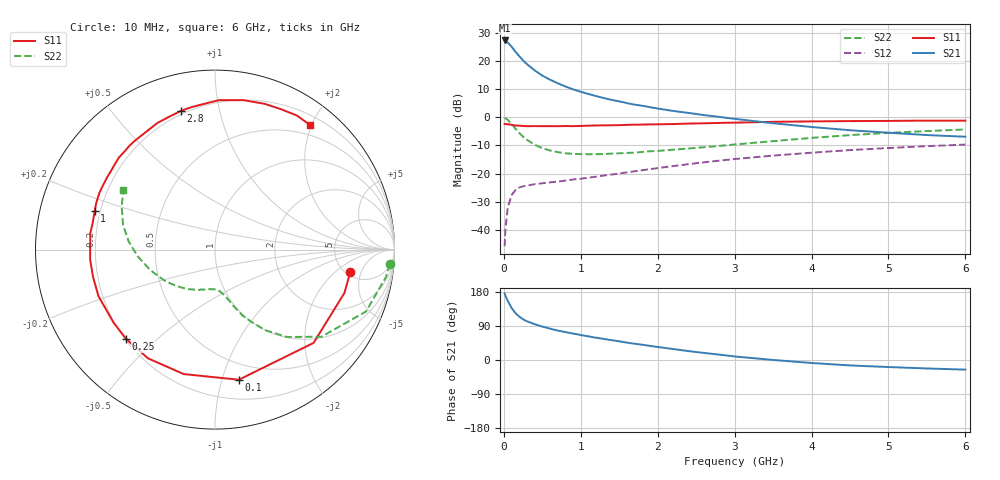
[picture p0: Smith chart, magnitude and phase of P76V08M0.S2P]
! SIEMENS Small Signal Semiconductors
! BFP196
! Si NPN RF Bipolar Junction Transistor in SOT143
! VCE = 6 V  IC = 8 mA
! Common Emitter S-Parameters:  May  1996
# GHz  S  MA  R  50
!  f  S11  S21  S12  S22
! GHz  MAG  ANG  MAG  ANG  MAG  ANG  MAG  ANG
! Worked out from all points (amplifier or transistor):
!   36 points, 10 MHz to 6 GHz, reference 50 ohm
!   highest |S21| = 27.4 dB at 10 MHz (marker M1)
!   |S21| within 3 dB of that: start of sweep to 123.2 MHz
!   unconditionally stable (mu >= 1): 965.9 MHz to 3.225 GHz
!   at 250 MHz: K = 0.34, MSG = 22.4 dB, |S12| = -24.5 dB
!   at 1.4 GHz: K = 1.14, MAG = 11.1 dB, |S12| = -20.4 dB
!   at 6 GHz: K = 0.97, MSG = 1.4 dB, |S12| = -9.7 dB
!   S11 on the Smith chart (normalised r, x): 10 MHz: 5.46, -3.27; 100 MHz: 0.36, -1.14; 250 MHz: 0.20, -0.40; 1 GHz: 0.18, +0.15; 2.8 GHz: 0.18, +0.77; 6 GHz: 0.34, +1.97
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0.01  0.764 -9.4  23.36 175.9  0.0051 88.6  0.9781 -4.8
0.02  0.7605 -18.5  22.82 169.8  0.01 81.9  0.9642 -9.2
0.05  0.7563 -43.4  21.47 156.3  0.0245 68.3  0.9092 -22.3
0.1  0.7371 -79.6  18.21 137.6  0.0412 53.7  0.7663 -39.3
0.15  0.7151 -104.1  14.79 123.8  0.0507 43.7  0.6301 -50.6
0.2  0.7116 -121.6  12.29 114.6  0.0563 37.9  0.5298 -58.0
0.25  0.702 -134.8  10.28 107.4  0.0593 34.2  0.4518 -63.2
0.3  0.6964 -144.2  8.852 102.2  0.0611 32.1  0.3989 -67.3
0.4  0.6991 -158.2  6.865 94.5  0.0646 30.1  0.3258 -72.2
0.5  0.6965 -167.4  5.544 88.2  0.0671 29.6  0.2834 -75.6
0.6  0.698 -175.5  4.679 82.7  0.0697 30.3  0.2569 -78.8
0.7  0.6958 177.8  4.041 77.8  0.0718 31.8  0.2406 -81.9
0.8  0.7008 172.4  3.545 73.7  0.075 32.6  0.2299 -84.6
1  0.7041 162.4  2.849 65.9  0.0809 35.1  0.2218 -89.2
1.1  0.7111 158.5  2.6 62.3  0.0844 36.4  0.2209 -92.2
1.6  0.7337 139.4  1.79 45.8  0.105 40.7  0.2327 -106.8
2.2  0.7597 120.6  1.3 29.0  0.1358 41.3  0.2657 -123.8
2.8  0.796 103.8  1.019 14.2  0.1695 38.4  0.3103 -142.3
3.5  0.8328 88.6  0.785 0.1  0.2085 31.9  0.377 -162.1
4.5  0.858 71.2  0.59 -14.3  0.2615 21.2  0.4828 174.7
5.5  0.8752 58.6  0.484 -22.3  0.307 9.6  0.5707 155.6
6  0.8729 52.8  0.452 -25.4  0.3279 3.2  0.6087 147.2
